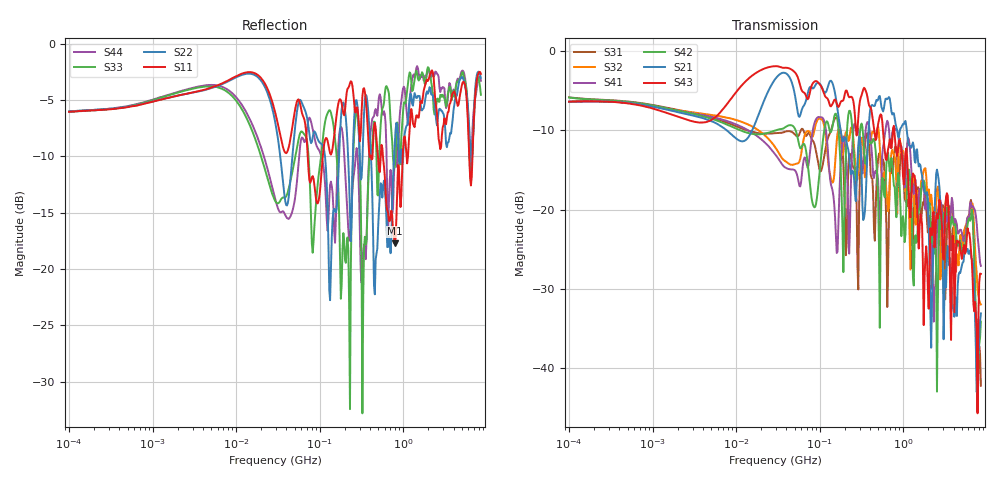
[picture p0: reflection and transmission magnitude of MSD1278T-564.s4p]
# MHz S MA R 50
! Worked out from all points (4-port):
!   498 points, 100 kHz to 8.5 GHz, reference 50 ohm
!   strongest paths, dB at 100 kHz, 1.698 MHz, 29.49 MHz, 500.7 MHz, 8.5 GHz:
!     S43: -6.4, -8.0, -1.9, -9.2, -28.1
!     S21: -6.4, -7.5, -3.5, -6.1, -33.1
!     S42: -5.8, -7.3, -10.0, -18.7, -34.1
!     S41: -6.4, -7.4, -13.0, -16.2, -27.1
!     S32: -6.4, -7.3, -12.1, -9.5, -31.9
!     S31: -5.8, -7.3, -10.3, -13.6, -42.2
!   lowest |S11| = -17.7 dB at 790.5 MHz (marker M1), VSWR 1.30, Z = 47.2 - j12.4 ohm
!   |S11| at or under -10 dB: 71.82 MHz to 108.9 MHz (37.07 MHz wide, 41 % of centre); 571.6 MHz to 986.7 MHz (415.2 MHz wide, 53.3 % of centre); 6.159 GHz to 6.738 GHz (578.4 MHz wide, 8.97 % of centre)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
0.1  0.4984 9.6  0.4802 7.9  0.5123 -10.5  0.4791 -173.4
     0.4802 7.9  0.5003 9.7  0.4789 -173.3  0.5105 -10.8
     0.5123 -10.5  0.4789 -173.3  0.4974 9.6  0.4807 7.8
     0.4791 -173.4  0.5105 -10.8  0.4807 7.8  0.4996 9.8
790.5161  0.1298 -95.3  0.3755 -112.2  0.2432 -70.1  0.3229 -83.5
          0.3755 -112.2  0.3561 -48.2  0.2175 -98.6  0.1384 -121.1
          0.2432 -70.1  0.2175 -98.6  0.2818 -74.7  0.2928 -131.4
          0.3229 -83.5  0.1384 -121.1  0.2928 -131.4  0.3216 -41.1
1367.575  0.4259 -126.8  0.2036 177.1  0.1272 -138.6  0.1462 -164.7
          0.2036 177.1  0.6037 -134.1  0.1021 -162.7  0.06278 -131.3
          0.1272 -138.6  0.1021 -162.7  0.6904 -127.3  0.1639 167.0
          0.1462 -164.7  0.06278 -131.3  0.1639 167.0  0.7083 -123.4
2713.323  0.3618 107.2  0.1382 45.0  0.07898 55.6  0.1148 118.5
          0.1382 45.0  0.5141 118.3  0.08047 36.3  0.09343 139.1
          0.07898 55.6  0.08047 36.3  0.5523 111.3  0.1156 76.7
          0.1148 118.5  0.09343 139.1  0.1156 76.7  0.6385 98.3
4802.421  0.5979 -83.7  0.03988 149.3  0.06758 -96.0  0.07485 -89.4
          0.03988 149.3  0.6948 -89.4  0.06906 -80.9  0.06423 -109.3
          0.06758 -96.0  0.06906 -80.9  0.6988 -99.0  0.05712 95.3
          0.07485 -89.4  0.06423 -109.3  0.05712 95.3  0.7138 -91.2
6462.473  0.2347 125.7  0.05108 1.0  0.1153 60.9  0.111 102.9
          0.05108 1.0  0.3034 141.9  0.1044 89.8  0.08762 75.0
          0.1153 60.9  0.1044 89.8  0.2422 85.8  0.05597 -83.6
          0.111 102.9  0.08762 75.0  0.05597 -83.6  0.2891 91.1
8500  0.7346 -55.1  0.02219 -29.8  0.007763 -95.5  0.04424 -134.7
      0.02219 -29.8  0.7046 -63.4  0.02528 178.4  0.01967 -74.6
      0.007763 -95.5  0.02528 178.4  0.5928 -63.8  0.0394 -49.1
      0.04424 -134.7  0.01967 -74.6  0.0394 -49.1  0.6844 -59.5
